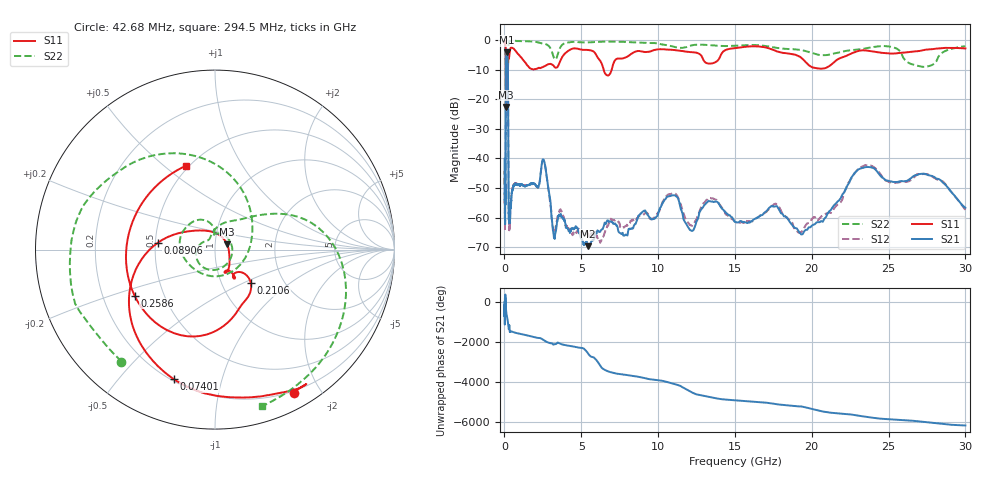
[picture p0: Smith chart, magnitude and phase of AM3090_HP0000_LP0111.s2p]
! Date/Time: Thu, Feb 28, 2019 1:53 PM
! Network Analyzer: Agilent Technologies E8364B Rev: A.07.50.67
! Sweep from 0.010 to 30.000 GHz, 1601 Points, Sweep Type: LOG
! Power Supply: 5.023 V, 0.002 A
# Hz S DB R 50
!freq MagS11 AngS11 MagS21 AngS21 MagS12 AngS12 MagS22 AngS22
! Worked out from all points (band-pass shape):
!   1601 points, 10 MHz to 30 GHz, reference 50 ohm
!   highest |S21| = -4.17 dB at 148.4 MHz (marker M1); lowest = -69.6 dB at 5.419 GHz (marker M2)
!   |S21| within 3 dB of the highest: 99.31 MHz to 216.5 MHz (117.2 MHz wide, 74.2 % of centre)
!   lowest |S11| = -22.6 dB at 97.46 MHz (marker M3), VSWR 1.16, Z = 57.1 + j3.39 ohm
!   |S11| at or under -10 dB: 89.17 MHz to 217.6 MHz (128.5 MHz wide, 83.8 % of centre); 6.454 GHz to 6.981 GHz (526.4 MHz wide, 7.84 % of centre)
!   |S22| runs from -23.8 to -0.2 dB; largest |S21 - S12| = 0.013
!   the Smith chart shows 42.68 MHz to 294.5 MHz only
!   S11 on the Smith chart (normalised r, x): 42.68 MHz: 0.17, -1.68; 74.01 MHz: 0.21, -0.71; 89.06 MHz: 0.51, +0.04; 210.6 MHz: 1.37, -0.55; 258.6 MHz: 0.34, -0.24; 294.5 MHz: 0.48, +0.60
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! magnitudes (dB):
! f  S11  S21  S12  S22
! 10 MHz  -0.3  -40.1  -49.0  -0.6
! 38.04 MHz  -0.5  -58.7  -63.4  -1.5
! 42.68 MHz  -0.8  -62.1  -60.8  -1.8
! 74.01 MHz  -2.4  -45.8  -45.9  -4.2
! 89.06 MHz  -9.8  -15.4  -15.4  -16.4
! 97.46 MHz  -22.6  -7.8  -7.8  -13.8
! 144.7 MHz  -15.0  -4.2  -4.1  -20.4
! 148.4 MHz  -14.9  -4.2  -4.1  -20.3
! 210.6 MHz  -11.3  -6.4  -6.3  -19.8
! 233.9 MHz  -8.1  -14.3  -14.2  -9.5
! 258.6 MHz  -5.7  -44.7  -44.3  -2.0
! 294.5 MHz  -6.1  -59.2  -60.6  -0.8
! 550.5 MHz  -2.8  -50.1  -49.8  -0.3
! 2.084 GHz  -9.8  -49.3  -49.5  -0.7
! 2.558 GHz  -9.0  -40.6  -40.5  -1.3
! 3.22 GHz  -8.9  -66.8  -64.7  -6.0
! 5.419 GHz  -3.4  -69.6  -65.3  -0.8
! 7.926 GHz  -5.9  -65.7  -62.8  -0.7
! 10.86 GHz  -3.3  -52.5  -51.9  -2.0
! 19.61 GHz  -7.5  -64.1  -62.5  -3.8
! 23.59 GHz  -3.6  -42.9  -42.3  -2.8
! 30 GHz  -2.9  -56.7  -57.4  -2.2
